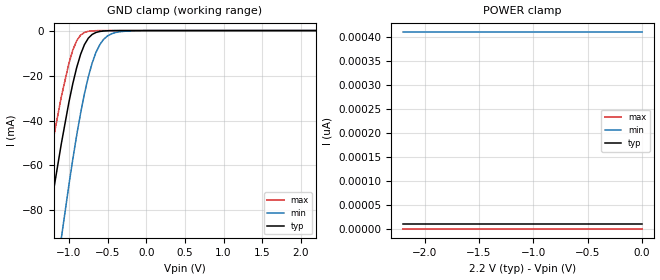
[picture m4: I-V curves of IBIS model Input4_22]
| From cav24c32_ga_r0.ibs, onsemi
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|//////////////////////////////////////////////////////////////////////////////
|//////////////////////////////////////////////////////////////////////////////
[Model]  Input4_22
Model_type Input
Vinh =  1.54
Vinl =  0.66
|  variable   typ   min   max
C_comp   6pF   NA   6pF
|//////////////////////////////////////////////////////////////////////////////
[Temperature Range]   25   NA   -40
|//////////////////////////////////////////////////////////////////////////////
[Voltage Range]   2.20V   NA   2.70V
|//////////////////////////////////////////////////////////////////////////////
[POWER Clamp Reference] 2.20V   NA   2.70V
|//////////////////////////////////////////////////////////////////////////////
[GND Clamp Reference]   0V   NA   0V
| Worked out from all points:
|   GND clamp passes 1 mA (typ) near -0.66 V on its own axis
|//////////////////////////////////////////////////////////////////////////////
[GND Clamp]
|   Voltage   I(typ)   I(min)   I(max)
-2.2V     -313mA     -411mA     -265mA
-1.4V     -116mA     -173mA     -88mA
-1.3V     -93.3mA    -145mA     -67.4mA
-1.2V     -71.2mA    -118mA     -47.7mA
-1.1V     -50.5mA    -92.6mA    -29.6mA
-950mV    -23.5mA    -57.1mA    -8.63mA
-900mV    -16.4mA    -46.5mA    -4.5mA
-800mV    -6.24mA    -28.1mA    -836uA
-700mV    -1.71mA    -14.4mA    -121uA
-600mV    -390uA     -6.16mA    -16.7uA
-400mV    -17.7uA    -880uA     -312nA
2.2V      10pA       409pA      12.9fA
|//////////////////////////////////////////////////////////////////////////////
[POWER Clamp]
|   Voltage   I(typ)   I(min)   I(max)
-2.2V     10pA       409pA      12.9fA
-2.1V     10pA       409pA      12.9fA
-2V       10pA       409pA      12.9fA
0V        10pA       409pA      12.9fA
